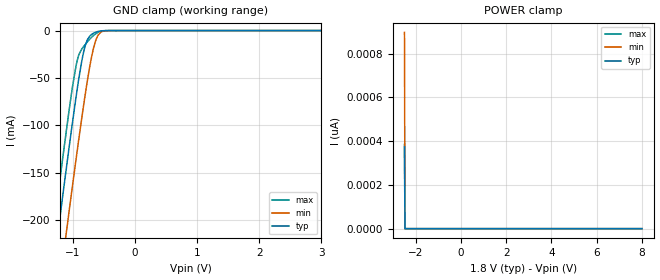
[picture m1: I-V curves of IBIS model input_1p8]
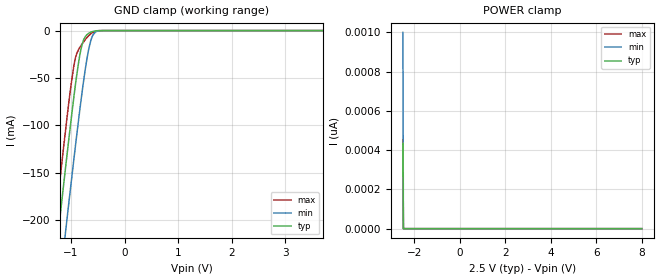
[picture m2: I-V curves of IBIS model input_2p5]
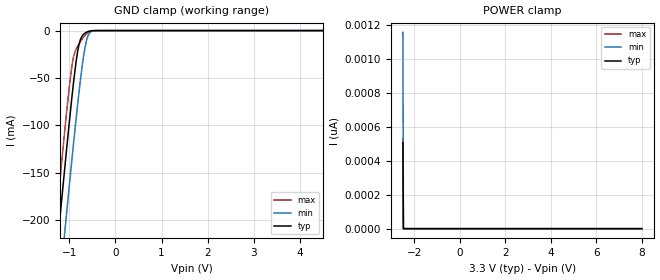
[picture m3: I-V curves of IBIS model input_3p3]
|Texas Instruments Incorporated
| Single Power Supply Single Buffer GATE with 3-State Output CMOS Logic
| Level Shifter
| Marketing part#   Digital Voltage Range   Package-type   #pins
| LV1T34QDBVRQ1   1.6V-5.5V   SOT-23   5
| LV1T34QDCKRQ1   1.6V-5.5V   SC70   5
[IBIS Ver]   4.1
[File name]   sn74lv1t34-q1.ibs
[File Rev]   1.0
[Date]   4/27/2022
[Source]
| Texas Instruments Incorporated.
| Analog-eLab Design Center, HPA
| 12500 TI Blvd
| Dallas, TX -75243
[Notes]   Revision History:
| Rev 1.0: 4/27/202-2
| - Model based on parent device LV1T34.
| - C_comp although listed in numerical order of value are
|   obtained from varying PVT conditions. For PVT conditions for
|   each specific value refer the buffer description under
|   respective [Model]. IBIS model user is responsible for using
|   appropriate C_comp to simulate for Signal Integrity.
[Disclaimer]
| This model is designed as an aid for customers of Texas Instruments.
| TI and its licensors and suppliers make no warranties, either expressed
| or implied, with respect to this  model, including the warranties of
| merchantability or fitness for a particular purpose. The model is
| provided solely on an "as is" basis. The entire risk as to its quality
| and performance is with the customer.
[Copyright]
(C) Copyright 2022 Texas Instruments Incorporated.All rights reserved.
|   SN74LV1T34QDBV
[Component]   SN74LV1T34QDBV
[Manufacturer]   TI
[Package]   |5 SOT-23  -  DBV package
|   typ   min   max
R_pkg   0.06209   0.05045   0.07001
L_pkg   1.83153nH   1.49378nH   2.04843nH
C_pkg   0.26256pF   0.24997pF   0.27952pF
[Pin]  signal_name   model_name   R_pin   L_pin   C_pin
1   NC   NC   0.07001   2.04843nH  0.27952pF
2   A   INPUT   0.05045   1.49378nH  0.25820pF
3   GND   GND   0.06850   2.45772nH  0.39635pF
4   Y   OUTPUT   0.06582   1.95239nH  0.24997pF
5   VCC   POWER   0.06589   1.95370nH  0.25029pF
|   SN74LV1T34DCK
[Component]   SN74LV1T34QDCK
[Manufacturer]   TI
[Package]   |5 SC70   -  DCK package
|   typ   min   max
R_pkg   0.04747   0.04577   0.04900
L_pkg   1.58367nH   1.46085nH   1.66427nH
C_pkg   0.23613pF   0.22997pF   0.24076pF
[Pin]  signal_name   model_name   R_pin   L_pin   C_pin
1   NC   NC   0.04900   1.62590nH  0.24076pF
2   A   INPUT   0.04577   1.46085nH  0.23766pF
3   GND   GND   0.04635   1.67071nH  0.26247pF
4   Y   OUTPUT   0.04763   1.66427nH  0.22997pF
5   VCC   POWER   0.04778   1.66679nH  0.23019pF
|   Model Selectors
[Model Selector] INPUT
input_1p8   1.8V  digital input
input_2p5   2.5V  digital input
input_3p3   3.3V  digital input
input_5   5.0V  digital input
[Model Selector] OUTPUT
output_1p8   1.8V  digital 3-state
output_2p5   2.5V  digital 3-state
output_3p3   3.3V  digital 3-state
output_5   5.0V  digital 3-state
| Models and submodels in the file (8): input_1p8 (Input), input_2p5 (Input), input_3p3 (Input), input_5 (Input), output_1p8 (Output), output_2p5 (Output), output_3p3 (Output), output_5 (Output)
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|   input_1p8 Model
[Model]   input_1p8
Model_type   Input
Vinl = 0.54
Vinh = 1.26
|   typ   min   max
C_comp   2.237pF   2.352pF   2.216pF
[Voltage Range]   1.8   1.65   1.95
[Temperature Range]   27   125   -40
[Power Clamp Reference]   1.8   1.65   1.95
[GND Clamp Reference]   0   0   0
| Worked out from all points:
|   GND clamp passes 1 mA (typ) near -0.59 V on its own axis
[GND Clamp]
|   Voltage   I(typ)   I(min)   I(max)
-2.5V     -886.1mA   -950.4mA   -849.8mA
-1.313V   -253.8mA   -321.8mA   -214mA
-1.23V    -210.5mA   -278.6mA   -170.6mA
-1.135V   -162.5mA   -230.4mA   -122.8mA
-1.072V   -131.1mA   -198.7mA   -91.82mA
-946mV    -70.84mA   -136.6mA   -37.84mA
-830.5mV  -25.02mA   -82.37mA   -17.55mA
-767.5mV  -10.52mA   -55.08mA   -12.35mA
-694mV    -4.055mA   -27.68mA   -6.988mA
-599.5mV  -1.104mA   -5.98mA    -2.17mA
-431.5mV  -13.53uA   -85.65uA   -11.55uA
8V        0A         0A         0A
[POWER Clamp]
|   Voltage   I(typ)   I(min)   I(max)
-2.5V     373.9pA    897.3pA    385.2pA
-2.479V   0A         0A         0A
-2.469V   0A         0A         0A
8V        0A         0A         0A
[Model]   input_2p5
Model_type   Input
Vinl = 0.75
Vinh = 1.75
|   typ   min   max
C_comp   2.237pF   2.352pF   2.216pF
[Voltage Range]   2.5   2.25   2.75
[Temperature Range]   27   125   -40
[Power Clamp Reference]   2.5   2.25   2.75
[GND Clamp Reference]   0   0   0
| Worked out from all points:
|   GND clamp passes 1 mA (typ) near -0.59 V on its own axis
[GND Clamp]
|   Voltage   I(typ)   I(min)   I(max)
-2.5V     -886.1mA   -950.4mA   -849.8mA
-1.313V   -253.8mA   -321.8mA   -214mA
-1.23V    -210.5mA   -278.6mA   -170.6mA
-1.135V   -162.5mA   -230.4mA   -122.8mA
-1.072V   -131.1mA   -198.7mA   -91.82mA
-946mV    -70.84mA   -136.6mA   -37.84mA
-830.5mV  -25.02mA   -82.37mA   -17.55mA
-767.5mV  -10.52mA   -55.08mA   -12.35mA
-694mV    -4.055mA   -27.68mA   -6.988mA
-599.5mV  -1.104mA   -5.98mA    -2.17mA
-431.5mV  -13.53uA   -85.65uA   -11.55uA
8V        0A         0A         0A
[POWER Clamp]
|   Voltage   I(typ)   I(min)   I(max)
-2.5V     435.2pA    1nA        455.2pA
-2.479V   0A         0A         0A
-2.469V   0A         0A         0A
8V        0A         0A         0A
[Model]   input_3p3
Model_type   Input
Vinl = 0.99
Vinh = 2.31
|   typ   min   max
C_comp   2.237pF   2.352pF   2.216pF
[Voltage Range]   3.3   3   3.6
[Temperature Range]   27   125   -40
[Power Clamp Reference]   3.3   3   3.6
[GND Clamp Reference]   0   0   0
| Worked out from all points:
|   GND clamp passes 1 mA (typ) near -0.59 V on its own axis
[GND Clamp]
|   Voltage   I(typ)   I(min)   I(max)
-2.5V     -886.1mA   -950.4mA   -849.8mA
-1.313V   -253.8mA   -321.8mA   -214mA
-1.23V    -210.5mA   -278.6mA   -170.6mA
-1.135V   -162.5mA   -230.4mA   -122.8mA
-1.072V   -131.1mA   -198.7mA   -91.82mA
-946mV    -70.84mA   -136.6mA   -37.84mA
-830.5mV  -25.02mA   -82.37mA   -17.55mA
-767.5mV  -10.52mA   -55.08mA   -12.35mA
-694mV    -4.055mA   -27.68mA   -6.988mA
-599.5mV  -1.104mA   -5.98mA    -2.17mA
-431.5mV  -13.53uA   -85.65uA   -11.55uA
8V        0A         0A         0A
[POWER Clamp]
|   Voltage   I(typ)   I(min)   I(max)
-2.5V     506pA      1.154nA    530.9pA
-2.479V   0A         0A         0A
-2.469V   0A         0A         0A
8V        0A         0A         0A
